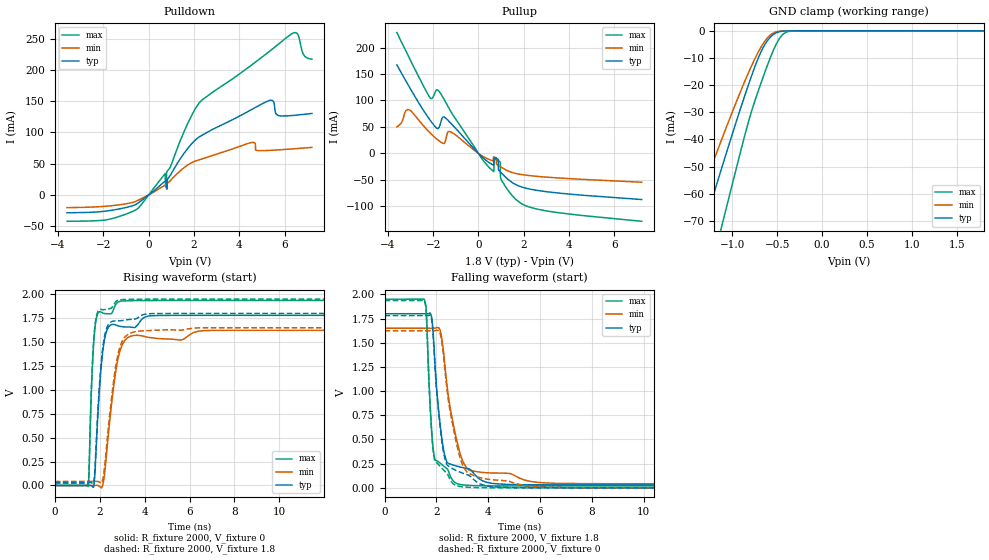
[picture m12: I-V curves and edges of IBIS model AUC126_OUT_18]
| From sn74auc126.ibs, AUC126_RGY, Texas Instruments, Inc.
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[Model]   AUC126_OUT_18
Model_type  3-state
Enable   Active-High
Vref =   0
Rref =   2000
Cref =   15p
Vmeas =   0.9
| variable   typ   min   max
C_comp   5.17pF   4.62pF   5.42pF
| C_pullup   5.90pF   1.36pF   12.77pF
| C_pulldown   6.43pF   5.22pF   15.40pF
| C_tri-state   5.17pF   4.62pF   5.42pF
[Temperature Range]   40   100   -40
| Ambient temperature   25   85   -40
[Voltage range]   1.8   1.65   1.95
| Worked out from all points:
|   slope of the pulldown table from 0 to 0.27 V, typ, clamps not added: 34.3 ohm
|   slope of the pullup table from 0 to 0.27 V, typ, clamps not added: 24.9 ohm
|   GND clamp passes 1 mA (typ) near -0.53 V on its own axis
|   rising waveform, R_fixture 2000, V_fixture 0: 20-80 % time 311ps typ, 490ps min, 196ps max; typ from 0 V to 1.78 V
|   falling waveform, R_fixture 2000, V_fixture 1.8: 20-80 % time 374ps typ, 601ps min, 226ps max; typ from 1.8 V to 0.031 V
|   rising waveform, R_fixture 2000, V_fixture 1.8: 20-80 % time 309ps typ, 486ps min, 194ps max; typ from 0.031 V to 1.8 V
|   falling waveform, R_fixture 2000, V_fixture 0: 20-80 % time 373ps typ, 598ps min, 226ps max; typ from 1.78 V to 0 V
[GND Clamp]
| AUC126_OUT_18
|   Voltage   I(typ)   I(min)   I(max)
-3.6V     -324.8mA   -272.6mA   -395.3mA
-1.48V    -89.78mA   -72.17mA   -119.8mA
-1.435V   -84.84mA   -68.08mA   -113.9mA
-1.3V     -70.1mA    -55.95mA   -96.04mA
-1.105V   -49.1mA    -38.82mA   -70.28mA
-830mV    -20.77mA   -16.17mA   -34.67mA
-685mV    -8.07mA    -6.262mA   -19.65mA
-565mV    -1.967mA   -1.239mA   -8.908mA
-490mV    -465.2uA   -242.6uA   -3.617mA
-425mV    -91.43uA   -52.01uA   -990.1uA
-300mV    -2.28uA    -2.125uA   -16.99uA
1.8V      471.3pA    37.67nA    526.5pA
[Pulldown]
| AUC126_OUT_18
|   Voltage   I(typ)   I(min)   I(max)
-3.6V     -28.49mA   -20.22mA   -42.08mA
-710mV    -17.24mA   -11.96mA   -26.36mA
730mV     22.14mA    15.83mA    34.29mA
740mV     22.44mA    16.07mA    13.19mA
780mV     23.67mA    17.08mA    13.96mA
805mV     10.91mA    9.302mA    37.17mA
2.235V    92.94mA    56.27mA    147.4mA
4.56V     137mA      84.03mA    208.3mA
5.345V    151.3mA    71.35mA    230.2mA
5.665V    128.2mA    72.04mA    239.5mA
6.27V     126.9mA    73.54mA    256.8mA
7.2V      130.4mA    76.05mA    217.2mA
[Pullup]
| AUC126_OUT_18
|   Voltage   I(typ)   I(min)   I(max)
-3.6V     167.2mA    50.11mA    228.2mA
-3.065V   126.7mA    82.61mA    181.6mA
-2.125V   62.44mA    38.39mA    104.7mA
-1.87V    48.93mA    28.24mA    118.8mA
-1.475V   67.8mA     21.29mA    99mA
-1.235V   57.67mA    40.84mA    80.46mA
395mV     -15.07mA   -10.01mA   -23mA
870mV     -11.11mA   -22.27mA   -13.48mA
955mV     -34.36mA   -24.54mA   -15.75mA
1.01V     -36.76mA   -26.02mA   -49.97mA
1.755V    -60.96mA   -38.77mA   -90.45mA
7.2V      -86.99mA   -54.32mA   -128.1mA
[Ramp]
| AUC126_OUT_18
| variable   typ   min   max
dV/dt_r   1.08/3.13E-10   0.99/4.98E-10   1.17/1.97E-10
dV/dt_f   1.07/3.76E-10   0.97/6.07E-10   1.16/2.31E-10
R_load = 2000
[Rising Waveform]
| AUC126_OUT_18
R_fixture =   2000
C_fixture =   0
L_fixture =   0
V_fixture =   0
V_fixture_min = 0
V_fixture_max = 0
|   Time   V(typ)   V(min)   V(max)
0s        8.422nV    29.16nV    1.154nV
1.48ns    116.7uV    -7.616uV   -11.63mV
1.52ns    249.7uV    -10.02uV   99mV
1.725ns   -18.73mV   208.6uV    1.465V
1.88ns    567.6mV    718.9uV    1.777V
2.185ns   1.489V     66.78mV    1.801V
2.855ns   1.668V     1.366V     1.923V
3.41ns    1.657V     1.565V     1.934V
6.605ns   1.78V      1.62V      1.936V
20ns      1.78V      1.624V     1.936V
[Falling Waveform]
| AUC126_OUT_18
R_fixture =   2000
C_fixture =   0
L_fixture =   0
V_fixture =   1.8
V_fixture_min = 1.65
V_fixture_max = 1.95
|   Time   V(typ)   V(min)   V(max)
0s        1.8V       1.65V      1.95V
1.535ns   1.8V       1.65V      1.945V
1.61ns    1.8V       1.65V      1.819V
1.81ns    1.773V     1.649V     620mV
1.92ns    1.406V     1.65V      321.9mV
2.295ns   371.3mV    1.358V     221.9mV
2.815ns   222.4mV    457.4mV    42.37mV
3.265ns   195.5mV    184.4mV    25.67mV
5.935ns   31.67mV    56.11mV    19.59mV
20ns      30.97mV    42.25mV    19.49mV
[Rising Waveform]
| AUC126_OUT_18
R_fixture =   2000
C_fixture =   0
L_fixture =   0
V_fixture =   1.8
V_fixture_min = 1.65
V_fixture_max = 1.95
|   Time   V(typ)   V(min)   V(max)
0s        30.94mV    42.24mV    19.47mV
1.48ns    31.05mV    42.23mV    8.483mV
1.52ns    31.18mV    42.23mV    124.3mV
1.62ns    30.36mV    42.23mV    955mV
1.725ns   17.37mV    42.44mV    1.489V
1.875ns   590.8mV    42.96mV    1.793V
2.17ns    1.498V     107.5mV    1.839V
2.805ns   1.722V     1.364V     1.937V
3.845ns   1.778V     1.617V     1.949V
20ns      1.8V       1.65V      1.95V
[Falling Waveform]
| AUC126_OUT_18
R_fixture =   2000
C_fixture =   0
L_fixture =   0
V_fixture =   0
V_fixture_min = 0
V_fixture_max = 0
|   Time   V(typ)   V(min)   V(max)
0s        1.78V      1.624V     1.936V
1.535ns   1.78V      1.624V     1.931V
1.61ns    1.78V      1.624V     1.804V
1.81ns    1.751V     1.623V     601.2mV
1.92ns    1.377V     1.623V     302.8mV
2.285ns   353.4mV    1.341V     181.9mV
2.79ns    176.2mV    439.7mV    21.97mV
3.24ns    130.6mV    152mV      6.073mV
5.66ns    924.8uV    15.05mV    132.4uV
20ns      33.01uV    9.226uV    13.36uV
